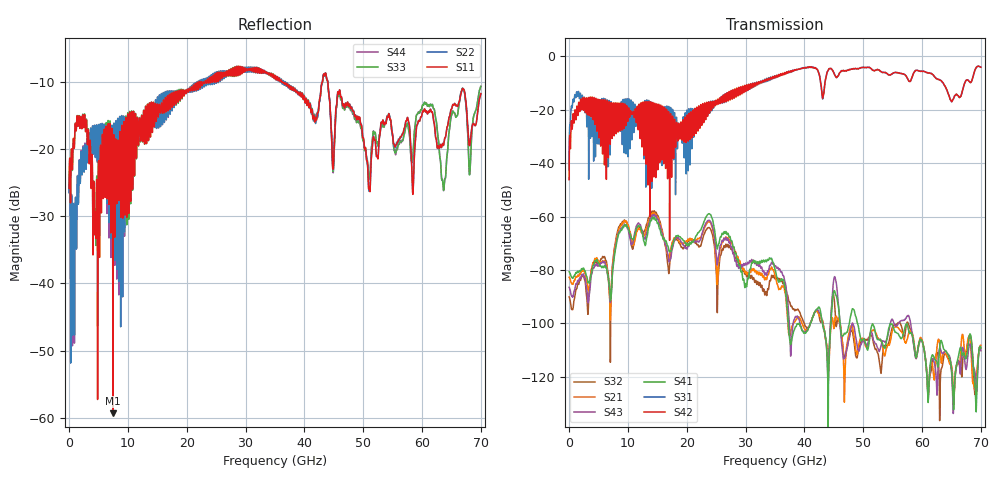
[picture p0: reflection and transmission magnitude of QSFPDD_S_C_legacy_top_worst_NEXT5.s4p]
! AWR Design Environment (8415) Fri Dec 21 09:21:28 2018
! Document = 'CHANNEL TEST'
! nPorts: 4, nXvals: 7001
# HZ S DB R 50
!Freq DBS11 AngS11 DBS12 AngS12 DBS13 AngS13 DBS14 AngS14
!	DBS21 AngS21 DBS22 AngS22 DBS23 AngS23 DBS24 AngS24
!	DBS31 AngS31 DBS32 AngS32 DBS33 AngS33 DBS34 AngS34
!	DBS41 AngS41 DBS42 AngS42 DBS43 AngS43 DBS44 AngS44
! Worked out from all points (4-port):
!   7000 points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, 10 MHz to 70 GHz, reference 50 ohm
!   strongest paths, dB at 10 MHz, 17.51 GHz, 35.01 GHz, 52.51 GHz, 70 GHz:
!     S42: -46.2, -25.1, -7.4, -5.0, -4.0
!     S31: -42.4, -23.4, -7.5, -5.0, -4.0
!     S41: -80.6, -70.9, -79.8, -106.0, -109.2
!     S43: -86.4, -72.3, -78.6, -109.4, -110.2
!     S21: -82.7, -69.7, -82.1, -105.4, -108.2
!     S32: -90.0, -71.2, -83.1, -111.3, -109.2
!   lowest |S11| = -59.3 dB at 7.44 GHz (marker M1), VSWR 1.00, Z = 50.1 - j0.0606 ohm
!   |S11| at or under -10 dB: start of sweep to 22.09 GHz; 36.3 GHz to 43.07 GHz (6.77 GHz wide, 17.1 % of centre); 43.97 GHz to end of sweep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
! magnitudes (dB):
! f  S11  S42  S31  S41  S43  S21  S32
! 10 MHz  -25.8  -46.2  -42.4  -80.6  -86.4  -82.7  -90.0
! 1.3 GHz  -15.8  -19.0  -13.2  -81.1  -85.2  -82.7  -87.0
! 7.44 GHz  -59.3  -18.3  -18.1  -79.6  -79.1  -77.3  -76.9
! 23.79 GHz  -9.6  -19.0  -17.2  -58.9  -61.3  -61.8  -64.1
! 29.49 GHz  -7.8  -11.3  -12.2  -82.8  -78.7  -79.5  -80.2
! 63.65 GHz  -19.4  -10.2  -10.2  -109.5  -111.1  -110.8  -112.9
! 70 GHz  -11.8  -4.0  -4.0  -109.2  -110.2  -108.2  -109.2
